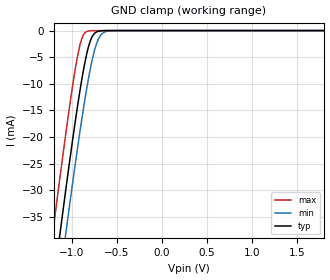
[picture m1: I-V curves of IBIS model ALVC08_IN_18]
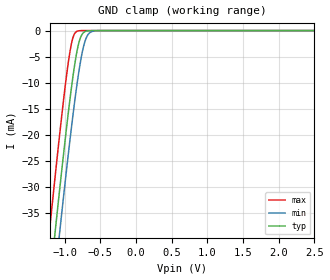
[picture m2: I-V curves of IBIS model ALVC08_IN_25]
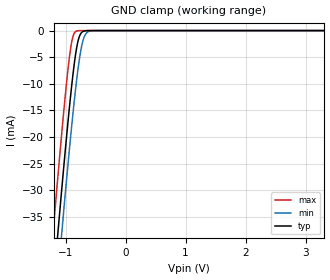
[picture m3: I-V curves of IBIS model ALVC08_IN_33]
| TEXAS INSTRUMENTS INCORPORATED
| Standard Linear and Logic Group
| IBIS Model of SN74ALVC08
| QUADRUPLE 2-INPUT POSITIVE-AND GATE
| This file contains package information for the following:
|  SOP 14-pin (NS) package as [Component] ALVC08_NS
|  TVSOP 14-pin (DGV) package as [Component] ALVC08_DGV
|  SOIC 14-pin (D) package as [Component] ALVC08_D
|  TSSOP 14-pin (PW) package as [Component] ALVC08_PW
|  QFN 14-pin (RGY) package as [Component] ALVC08_RGY
| This device can be powered at the following Vccs:
|  1.8 volt Vcc
|  2.5 volt Vcc
|  3.3 volt Vcc
| This file provides unique models under the [Model Selector] for each Vcc.
| For operation at a specific Vcc, select the appropriate model after each
| [Model Selector] keyword.
[IBIS Ver]   3.2
[Comment char]  |_char
[File Name]   sn74alvc08.ibs
[File Rev]   1.2 | a_die
[Date]   April 13, 2004
[Source]   Data created from TI-SPICE simulations at TI-SLL.
[Notes]   The following is an IBIS list for the ALVC08.
   Please contact sllibis@ti.com with questions and
   comments concerning SLL IBIS models.
   - FILE REV HISTORY
   - 1.2 RGY package added to IBIS file on 04/13/04
   - C_comp values are taken at a different test condition
   than the data sheet.
   - Power clamp data deleted as there is no power-clamp diode.
[Disclaimer] Property of Texas Instruments Incorporated.  Unauthorized
   reproduction and/or distribution is strictly prohibited.
   This product is protected under copyright law.
   Created  2002, (C) Copyright  2002, Texas Instruments
   Incorporated, All Rights Reserved
   UNLESS THERE IS A SIGNED, WRITTEN AGREEMENT TO THE
   CONTRARY, TEXAS INSTRUMENTS (TI) IS PROVIDING THE IBIS
   MODELS  AND WITHOUT ANY WARRANTY, EXPRESSED OR
   IMPLIED.  TI assumes no liability for:
   1) the accuracy of the IBIS models provided to your
   company;
   2) the proper functioning of these IBIS Models in your
   design or for any resulting applications; or
   3) infringement of patents, copyrights or intellectual
   property rights resulting from your use of these IBIS
   models.
   TI provides IBIS Models as a service to our customers.
   You and your company shall not distribute, sell or give
   these models to anyone else without prior written
   permission from TI.
   TI reserves the right to make changes to our products or
   to discontinue any semiconductor product or service
   without notice, and advises our customers to obtain the
   latest version of relevant information to verify, before
   placing orders, that the information being relied on is
   current.
   Please be aware that your receipt and use of the IBIS
   information provided shall serve as acceptance of these
   terms and conditions.  If you do not accept these terms,
   you should return or destroy the IBIS models and any
   other accompanying information immediately.
| Component ALVC08_NS 14-pin SOP
[Component]   ALVC08_NS
[Manufacturer]  Texas Instruments, Inc.
[Package]
|   typ   min   max
R_pkg   4.500e-02   3.900e-02   5.400e-02
L_pkg   3.796e-09   2.561e-09   4.952e-09
C_pkg   5.280e-13   2.880e-13   7.100e-13
[Pin]   signal_name   model_name   R_pin   L_pin   C_pin
1   1A   ALVC08_IN   4.700e-02   4.867e-09   7.060e-13
2   1B   ALVC08_IN   5.100e-02   4.083e-09   5.920e-13
3   1Y   ALVC08_OUT   4.100e-02   2.915e-09   3.760e-13
4   2A   ALVC08_IN   3.900e-02   2.561e-09   2.880e-13
5   2B   ALVC08_IN   4.100e-02   3.101e-09   4.300e-13
6   2Y   ALVC08_OUT   4.700e-02   4.047e-09   5.890e-13
7   GND   GND   5.100e-02   4.909e-09   7.000e-13
8   3Y   ALVC08_OUT   4.500e-02   4.784e-09   6.940e-13
9   3A   ALVC08_IN   5.400e-02   4.176e-09   5.970e-13
10   3B   ALVC08_IN   3.900e-02   3.287e-09   4.490e-13
11   4Y   ALVC08_OUT   3.900e-02   2.586e-09   2.940e-13
12   4A   ALVC08_IN   4.000e-02   2.802e-09   3.710e-13
13   4B   ALVC08_IN   4.900e-02   4.080e-09   5.930e-13
14   VCC   POWER   5.200e-02   4.952e-09   7.100e-13
| Component ALVC08_DGV 14-pin TVSOP
[Component]   ALVC08_DGV
[Manufacturer]  Texas Instruments, Inc.
[Package]
|   typ   min   max
R_pkg   3.500e-02   2.000e-02   4.500e-02
L_pkg   2.499e-09   2.077e-09   2.966e-09
C_pkg   3.610e-13   3.050e-13   4.160e-13
[Pin]   signal_name   model_name   R_pin   L_pin   C_pin
1   1A   ALVC08_IN   2.700e-02   2.717e-09   3.730e-13
2   1B   ALVC08_IN   3.700e-02   2.434e-09   3.980e-13
3   1Y   ALVC08_OUT   3.400e-02   2.200e-09   3.160e-13
4   2A   ALVC08_IN   2.000e-02   2.077e-09   3.090e-13
5   2B   ALVC08_IN   3.000e-02   2.147e-09   3.050e-13
6   2Y   ALVC08_OUT   4.200e-02   2.580e-09   4.080e-13
7   GND   GND   3.900e-02   2.921e-09   3.850e-13
8   3Y   ALVC08_OUT   3.300e-02   2.841e-09   3.800e-13
9   3A   ALVC08_IN   4.200e-02   2.611e-09   4.100e-13
10   3B   ALVC08_IN   3.800e-02   2.331e-09   3.290e-13
11   4Y   ALVC08_OUT   2.600e-02   2.223e-09   3.190e-13
12   4A   ALVC08_IN   3.400e-02   2.259e-09   3.130e-13
13   4B   ALVC08_IN   4.500e-02   2.681e-09   4.160e-13
14   VCC   POWER   4.200e-02   2.966e-09   3.860e-13
| Component ALVC08_D 14-pin SOIC
[Component]   ALVC08_D
[Manufacturer]  Texas Instruments, Inc.
[Package]
|   typ   min   max
R_pkg   3.100e-02   2.800e-02   3.400e-02
L_pkg   3.109e-09   2.462e-09   3.889e-09
C_pkg   4.730e-13   3.630e-13   6.280e-13
[Pin]   signal_name   model_name   R_pin   L_pin   C_pin
1   1A   ALVC08_IN   3.300e-02   3.854e-09   6.220e-13
2   1B   ALVC08_IN   3.200e-02   3.188e-09   4.730e-13
3   1Y   ALVC08_OUT   2.800e-02   2.462e-09   3.770e-13
4   2A   ALVC08_IN   3.100e-02   2.596e-09   3.630e-13
5   2B   ALVC08_IN   2.800e-02   2.521e-09   3.720e-13
6   2Y   ALVC08_OUT   3.400e-02   3.250e-09   4.760e-13
7   GND   GND   3.400e-02   3.889e-09   6.280e-13
8   3Y   ALVC08_OUT   3.400e-02   3.889e-09   6.280e-13
9   3A   ALVC08_IN   3.400e-02   3.250e-09   4.760e-13
10   3B   ALVC08_IN   2.800e-02   2.521e-09   3.720e-13
11   4Y   ALVC08_OUT   3.100e-02   2.596e-09   3.640e-13
12   4A   ALVC08_IN   2.800e-02   2.462e-09   3.770e-13
13   4B   ALVC08_IN   3.200e-02   3.188e-09   4.730e-13
14   VCC   POWER   3.300e-02   3.854e-09   6.220e-13
| Component ALVC08_PW 14-pin TSSOP
[Component]   ALVC08_PW
[Manufacturer]  Texas Instruments, Inc.
[Package]
|   typ   min   max
R_pkg   3.200e-02   2.900e-02   3.500e-02
L_pkg   2.378e-09   2.170e-09   2.680e-09
C_pkg   3.140e-13   2.700e-13   3.350e-13
[Pin]   signal_name   model_name   R_pin   L_pin   C_pin
1   1A   ALVC08_IN   3.300e-02   2.618e-09   3.300e-13
2   1B   ALVC08_IN   3.100e-02   2.313e-09   3.170e-13
3   1Y   ALVC08_OUT   3.000e-02   2.310e-09   3.140e-13
4   2A   ALVC08_IN   3.100e-02   2.173e-09   2.720e-13
5   2B   ALVC08_IN   3.000e-02   2.204e-09   3.090e-13
6   2Y   ALVC08_OUT   3.200e-02   2.315e-09   3.170e-13
7   GND   GND   3.500e-02   2.680e-09   3.350e-13
8   3Y   ALVC08_OUT   3.300e-02   2.640e-09   3.330e-13
9   3A   ALVC08_IN   3.400e-02   2.347e-09   3.190e-13
10   3B   ALVC08_IN   2.900e-02   2.277e-09   3.130e-13
11   4Y   ALVC08_OUT   3.100e-02   2.170e-09   2.700e-13
12   4A   ALVC08_IN   3.100e-02   2.244e-09   3.110e-13
13   4B   ALVC08_IN   3.300e-02   2.343e-09   3.210e-13
14   VCC   POWER   3.500e-02   2.657e-09   3.320e-13
| Component ALVC08_RGY 14-pin QFN
[Component]   ALVC08_RGY
[Manufacturer]   Texas Instruments, Inc.
[Package]
|   typ   min   max
R_pkg   2.900e-02   2.300e-02   4.100e-02
L_pkg   7.730e-10   6.570e-10   9.980e-10
C_pkg   1.360e-13   1.150e-13   1.560e-13
[Pin]   signal_name   model_name   R_pin   L_pin   C_pin
1   1A   ALVC08_IN   2.700e-02   8.310e-10   1.300e-13
2   1B   ALVC08_IN   2.700e-02   8.660e-10   1.350e-13
3   1Y   ALVC08_OUT   4.100e-02   9.980e-10   1.560e-13
4   2A   ALVC08_IN   3.100e-02   7.670e-10   1.420e-13
5   2B   ALVC08_IN   3.100e-02   7.650e-10   1.420e-13
6   2Y   ALVC08_OUT   3.100e-02   7.830e-10   1.440e-13
7   GND   GND   3.100e-02   7.810e-10   1.370e-13
8   3Y   ALVC08_OUT   2.300e-02   6.570e-10   1.150e-13
9   3A   ALVC08_IN   2.300e-02   8.140e-10   1.290e-13
10   3B   ALVC08_IN   2.800e-02   7.040e-10   1.290e-13
11   4Y   ALVC08_OUT   2.700e-02   6.720e-10   1.360e-13
12   4A   ALVC08_IN   2.700e-02   6.960e-10   1.380e-13
13   4B   ALVC08_IN   2.700e-02   7.250e-10   1.400e-13
14   VCC   POWER   3.000e-02   7.630e-10   1.360e-13
| Model ALVC08_IN
[Model Selector]   ALVC08_IN
ALVC08_IN_18   1.8 volt Vcc
ALVC08_IN_25   2.5 volt Vcc
ALVC08_IN_33   3.3 volt Vcc
| Model ALVC08_OUT
[Model Selector]   ALVC08_OUT
ALVC08_OUT_18   1.8 volt Vcc
ALVC08_OUT_25   2.5 volt Vcc
ALVC08_OUT_33   3.3 volt Vcc
| Models and submodels in the file (6): ALVC08_IN_18 (Input), ALVC08_IN_25 (Input), ALVC08_IN_33 (Input), ALVC08_OUT_18 (Output), ALVC08_OUT_25 (Output), ALVC08_OUT_33 (Output)
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[Model]   ALVC08_IN_18
Model_type  Input
Vinl=0.5775
Vinh=1.2675
| variable   typ   min   max
C_comp   3.95pF   3.44pF   4.64pF
[Temperature Range]   40   100   -40
| Ambient temperature   25   85   -40
[Voltage range]   1.8   1.65   1.95
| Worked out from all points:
|   GND clamp passes 1 mA (typ) near -0.77 V on its own axis
[GND Clamp]
| ALVC08_IN_18
|   Voltage   I(typ)   I(min)   I(max)
-1.8V     -129.8mA   -137.8mA   -119.7mA
-1.205V   -48.27mA   -56.56mA   -37.63mA
-1.125V   -37.77mA   -46.06mA   -27.13mA
-1.06V    -29.44mA   -37.69mA   -18.89mA
-980mV    -19.61mA   -27.69mA   -9.485mA
-925mV    -13.29mA   -21.11mA   -4.122mA
-880mV    -8.606mA   -15.99mA   -1.263mA
-835mV    -4.656mA   -11.25mA   -214.1uA
-780mV    -1.472mA   -6.227mA   -17.15uA
-725mV    -285.9uA   -2.596mA   -1.294uA
-615mV    -6.479uA   -167.8uA   -7.305nA
1.8V      3.326pA    6.142pA    3.026pA
[Model]   ALVC08_IN_25
Model_type  Input
Vinl=0.7
Vinh=1.7
| variable   typ   min   max
C_comp   3.89pF   3.12pF   4.62pF
[Temperature Range]   40   100   -40
| Ambient temperature   25   85   -40
[Voltage range]   2.5   2.3   2.7
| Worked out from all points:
|   GND clamp passes 1 mA (typ) near -0.77 V on its own axis
[GND Clamp]
| ALVC08_IN_25
|   Voltage   I(typ)   I(min)   I(max)
-2.5V     -228.1mA   -235.8mA   -218.5mA
-1.23V    -51.59mA   -59.87mA   -40.97mA
-1.2V     -47.61mA   -55.9mA    -36.97mA
-1.13V    -38.42mA   -46.71mA   -27.77mA
-1.07V    -30.71mA   -38.96mA   -20.13mA
-925mV    -13.29mA   -21.11mA   -4.122mA
-880mV    -8.606mA   -15.99mA   -1.263mA
-830mV    -4.281mA   -10.75mA   -171.6uA
-780mV    -1.472mA   -6.227mA   -17.15uA
-720mV    -242.5uA   -2.354mA   -1.023uA
-600mV    -3.832uA   -109.2uA   -3.608nA
2.5V      4.713pA    7.577pA    4.389pA
[Model]   ALVC08_IN_33
Model_type  Input
Vinl=0.8
Vinh=2.0
| variable   typ   min   max
C_comp   3.87pF   2.95pF   5.13pF
[Temperature Range]   40   100   -40
| Ambient temperature   25   85   -40
[Voltage range]   3.3   3   3.6
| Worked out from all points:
|   GND clamp passes 1 mA (typ) near -0.77 V on its own axis
[GND Clamp]
| ALVC08_IN_33
|   Voltage   I(typ)   I(min)   I(max)
-3.3V     -341.5mA   -348.9mA   -332.3mA
-1.215V   -49.6mA    -57.88mA   -38.96mA
-1.185V   -45.62mA   -53.91mA   -34.98mA
-1.125V   -37.77mA   -46.06mA   -27.13mA
-1.065V   -30.08mA   -38.33mA   -19.51mA
-920mV    -12.75mA   -20.53mA   -3.718mA
-875mV    -8.124mA   -15.45mA   -1.065mA
-825mV    -3.922mA   -10.26mA   -137.1uA
-775mV    -1.291mA   -5.83mA    -13.57uA
-715mV    -205.4uA   -2.128mA   -808.5nA
-585mV    -2.266uA   -70.82uA   -1.783nA
3.3V      6.304pA    9.258pA    5.93pA
